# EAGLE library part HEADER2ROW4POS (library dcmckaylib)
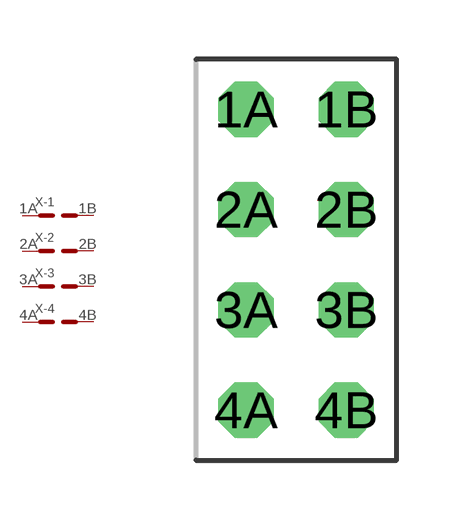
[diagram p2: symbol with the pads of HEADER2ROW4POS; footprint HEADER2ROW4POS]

Designator prefix X; gates -1=HEADER2ROW -2=HEADER2ROW -3=HEADER2ROW -4=HEADER2ROW

## HEADER2ROW4POS  [HEADER2ROW4POS]
1A  -1:P$1
1B  -1:P$2
2A  -2:P$1
2B  -2:P$2
3A  -3:P$1
3B  -3:P$2
4A  -4:P$1
4B  -4:P$2

## Footprint HEADER2ROW4POS (pad centres in mm)
drill 0.889 octagon: 1A -1.27,5.08; 1B 1.27,5.08; 2A -1.27,2.54; 2B 1.27,2.54; 3A -1.27,0; 3B 1.27,0; 4A -1.27,-2.54; 4B 1.27,-2.54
